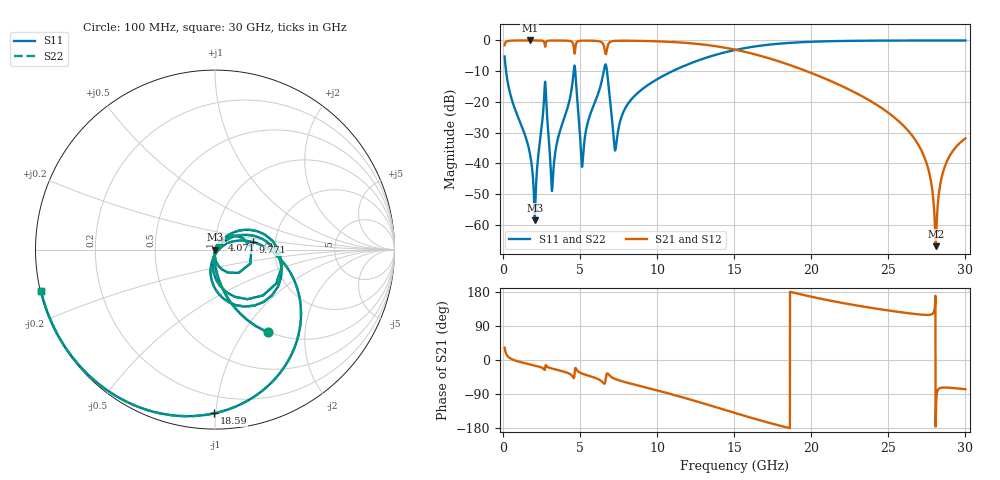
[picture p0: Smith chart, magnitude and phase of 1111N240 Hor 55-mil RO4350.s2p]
# GHz S MA R 50
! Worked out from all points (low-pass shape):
!   3201 points, 100 MHz to 30 GHz, reference 50 ohm
!   highest |S21| = -0.01 dB at 1.726 GHz (marker M1); lowest = -67.0 dB at 28.08 GHz (marker M2)
!   |S21| within 3 dB of the highest: start of sweep to 4.606 GHz; 6.735 GHz to 15.06 GHz (8.326 GHz wide, 76.4 % of centre)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
!   lowest |S11| = -58.6 dB at 2.062 GHz (marker M3), VSWR 1.00, Z = 50.1 - j0.0202 ohm
!   |S11| at or under -10 dB: 195.5 MHz to 4.581 GHz (4.385 GHz wide, 184 % of centre); 4.684 GHz to 6.533 GHz (1.849 GHz wide, 33 % of centre); 6.744 GHz to 10.99 GHz (4.249 GHz wide, 47.9 % of centre)
!   |S22| runs from -58.6 to 0.0 dB; largest |S21 - S12| = 0
!   S11 on the Smith chart (normalised r, x): 100 MHz: 0.98, -1.30; 4.071 GHz: 1.07, +0.11; 9.771 GHz: 1.53, +0.13; 18.59 GHz: 0.09, -0.99; 30 GHz: 0.00, -0.12
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0.1  0.5476 -57.5  0.8365 32.5  0.8365 32.5  0.5476 -57.5
1.725812  0.01514 -98.1  0.9988 -11.4  0.9988 -11.4  0.01514 -98.1
2.062187  0.00118 -9.8  0.9986 -14.7  0.9986 -14.7  0.00118 -9.8
2.688219  0.1529 28.6  0.9038 -26.2  0.9038 -26.2  0.1529 28.6
3.192781  0.003849 5.4  0.9962 -22.7  0.9962 -22.7  0.003849 5.4
4.071094  0.0649 53.7  0.993 -32.3  0.993 -32.3  0.0649 53.7
4.641063  0.3902 -29.0  0.6104 -34.7  0.6104 -34.7  0.3902 -29.0
5.089563  0.01083 -63.4  0.9899 -35.2  0.9899 -35.2  0.01083 -63.4
6.60325  0.3858 -15.9  0.6904 -61.5  0.6904 -61.5  0.3858 -15.9
7.294688  0.01672 -23.5  0.9842 -50.4  0.9842 -50.4  0.01672 -23.5
8.032844  0.08735 26.4  0.9892 -59.6  0.9892 -59.6  0.08735 26.4
9.770781  0.2159 11.1  0.9712 -77.8  0.9712 -77.8  0.2159 11.1
10.06978  0.2392 8.0  0.9657 -81.0  0.9657 -81.0  0.2392 8.0
15.05  0.6982 -50.2  0.708 -139.8  0.708 -139.8  0.6982 -50.2
18.59128  0.912 -90.2  0.3989 -179.8  0.3989 -179.8  0.912 -90.2
20.03956  0.9519 -103.8  0.2926 166.6  0.2926 166.6  0.9519 -103.8
25.01978  0.9945 -140.1  0.06594 130.6  0.06594 130.6  0.9945 -140.1
27.24359  0.9967 -152.7  0.01436 119.4  0.01436 119.4  0.9967 -152.7
27.71078  0.9968 -155.2  0.006026 119.4  0.006026 119.4  0.9968 -155.2
28.07519  0.9968 -157.1  0.0004486 -157.3  0.0004486 -157.3  0.9968 -157.1
28.68253  0.9968 -160.1  0.009113 -72.6  0.009113 -72.6  0.9968 -160.1
30  0.9965 -166.5  0.02547 -77.1  0.02547 -77.1  0.9965 -166.5
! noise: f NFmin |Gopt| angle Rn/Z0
0.1  0.0007086  0.7504  2.286  0.000572
3.417  0.01304  0.5833  23.98  0.005476
6.743  0.1995  0.9363  46.44  0.5902
10.06  0.02838  0.5035  63.6  0.007446
13.39  0.03876  0.5383  78.55  0.009446
16.7  0.05948  0.6413  94.51  0.01524
20.03  0.1048  0.7725  112.7  0.02993
23.35  0.2332  0.891  131.8  0.07907
26.67  1.068  0.9749  149.9  0.6589
30  1.083  0.9747  166.4  0.1403
